(* Logix 5000 AddOnInstructionDefinition export YAI_Assy_166_115_EIP_Hz; software revision 21.03 *)

ADD_ON_INSTRUCTION YAI_Assy_166_115_EIP_Hz   (* revision 1.0, vendor Yaskawa America, Inc. *)
// YAI Assembly 166 and 115
// Help:
// This add-on instruction is for use with input assemblie 166 and output assemblies 115.
// Node_Input_Assy is defined as the node's input assembly integer array.
// Node_Output_Assy is defined as the node's output assembly integer array.
// Torque limit/reference, torque compensation and torque output variables are only available with A1000.
VAR_IN_OUT
   Node_Input_Assy : AB:ETHERNET_MODULE_INT_44Bytes:I:0; {required}   // Input assembly words
   Node_Output_Assy : AB:ETHERNET_MODULE_INT_40Bytes:O:0; {required}   // Output assembly words
END_VAR
VAR_INPUT
   RunFwd : BOOL; {visible}   // Forward run command
   RunRev : BOOL; {visible}   // Reverse run command
   MFI_3 : BOOL; {visible}   // Multi-function input 3
   MFI_4 : BOOL; {visible}   // Multi-function input 4
   MFI_5 : BOOL; {visible}   // Multi-function input 5
   MFI_6 : BOOL; {visible}   // Multi-function input 6
   MFI_7 : BOOL; {visible}   // Multi-function input 7
   MFI_8 : BOOL; {visible}   // Multi-function input 8
   External_Fault : BOOL;   // External fault command (EF0)
   FaultReset : BOOL; {visible}   // Fault reset command
   MFO_1 : BOOL; {visible}   // Multi-function output (M1-M2 for A/P1000, MA/MB/MC for V1000)
   MFO_2 : BOOL; {visible}   // Multi-function output (M3-M4 for A/P1000, P1 for V1000)
   MFO_3 : BOOL; {visible}   // Multi-function output (M5-M6 for A/P1000, P2 for V1000)
   Freq_Ref : REAL; {visible}   // Frequency reference command in Hz (xx.xx resolution)
   Torq_Ref_Limit : REAL; {visible}   // Torque reference/limit (A1000 only)
   Torq_Comp : REAL; {visible}   // Torque compensation command (A1000 only)
   Analog_Output_1 : REAL;   // Analog output 1 level command
   Analog_Output_2 : REAL;   // Analog output 2 level command
   Digital_Output_1 : BOOL;   // Digital output 1 activation - M1-M2
   Digital_Output_2 : BOOL;   // Digital output 2 activation - M3-M4
   Digital_Output_3 : BOOL;   // Digital output 3 activation - M5-M6
   Digital_Output_Fault_Enable : BOOL;   // Bit to enable control of fault output relay over the network
   Digital_Output_Fault : BOOL;   // Fault relay activation - MA-MB-MC
END_VAR
VAR_OUTPUT
   Alarm : BOOL; {access Read Only, visible}   // Drive alarm status bit
   Analog_Input_1_Level : REAL; {access Read Only}   // Analog input 1 level in % (xxx.x resolution)
   At_Speed : BOOL; {access Read Only, visible}   // Drive at commanded speed status bit
   Custom_In_1 : INT; {access Read Only, visible}   // Custom input 1 - F7-33
   Custom_In_1_Error : BOOL; {access Read Only}   // Custom input 1 error bit
   Custom_In_2 : INT; {access Read Only, visible}   // Custom input 2 - F7-34
   Custom_In_2_Error : BOOL; {access Read Only}   // Custom input 2 error bit
   Custom_In_3 : INT; {access Read Only, visible}   // Custom input 3 - F7-35
   Custom_In_3_Error : BOOL; {access Read Only}   // Custom input 3 error bit
   Custom_In_4 : INT; {access Read Only}   // Custom input 4 - F7-36
   Custom_In_4_Error : BOOL; {access Read Only}   // Custom input 4 error bit
   Custom_In_5 : INT; {access Read Only}   // Custom input 5 - F7-37
   Custom_In_5_Error : BOOL; {access Read Only}   // Custom input 5 error bit
   Custom_In_6 : INT; {access Read Only}   // Custom input 6 - F7-38
   Custom_In_6_Error : BOOL; {access Read Only}   // Custom input 6 error bit
   Custom_In_7 : INT; {access Read Only}   // Custom input 7 - F7-39
   Custom_In_7_Error : BOOL; {access Read Only}   // Custom input 7 error bit
   Custom_In_8 : INT; {access Read Only}   // Custom input 8 -F7-40
   Custom_In_8_Error : BOOL; {access Read Only}   // Custom input 8 error bit
   Custom_In_9 : INT; {access Read Only}   // Custom input 9 - F7-41
   Custom_In_9_Error : BOOL; {access Read Only}   // Custom input 9 error bit
   Custom_In_10 : INT; {access Read Only}   // Custom input 10 - F7-42
   Custom_In_10_Error : BOOL; {access Read Only}   // Custom input 10 error bit
   Custom_Out_1_Error : BOOL; {access Read Only}   // Custom output 1 error bit
   Custom_Out_2_Error : BOOL; {access Read Only}   // Custom output 2 error bit
   Custom_Out_3_Error : BOOL; {access Read Only}   // Custom output 3 error bit
   Custom_Out_4_Error : BOOL; {access Read Only}   // Custom output 4 error bit
   Custom_Out_5_Error : BOOL; {access Read Only}   // Custom output 5 error bit
   Custom_Out_6_Error : BOOL; {access Read Only}   // Custom output 6 error bit
   Custom_Out_7_Error : BOOL; {access Read Only}   // Custom output 7 error bit
   Custom_Out_8_Error : BOOL; {access Read Only}   // Custom output 8 error bit
   Custom_Out_9_Error : BOOL; {access Read Only}   // Custom output 9 error bit
   Custom_Out_10_Error : BOOL; {access Read Only}   // Custom output 10 error bit
   DC_Bus_Volt : INT; {access Read Only, visible}   // DC bus voltage in Vdc (xxx resolution)
   Error_Code : INT; {access Read Only}   // Custom input/output error code. Refer to custom error bit to determine which parameter error is pertaining to.
   Faulted : BOOL; {access Read Only, visible}   // Drive faulted status bit
   Freq_Cmd : REAL; {access Read Only, visible}   // Commanded frequency in Hz (xx.xx resolution)
   MFO_1_Status : BOOL; {access Read Only, visible}   // Drive multi-function output 1 (M1-M2 for A/P1000, MA/MB/MC for V1000) status
   MFO_2_Status : BOOL; {access Read Only, visible}   // Drive multi-function output 1 (M3-M4 for A/P1000, P1 for V1000) status
   MFO_3_Status : BOOL; {access Read Only, visible}   // Drive multi-function output 1 (M5-M6 for A/P1000, P2 for V1000) status
   Motor_Speed : REAL; {access Read Only, visible}   // Motor speed in Hz (xx.xx resolution)
   NetCtrlStatus : BOOL; {access Read Only, visible}   // Drive network run source status bit (1 = source coming from network)
   OPE : BOOL; {access Read Only}   // OPE alarm/fault present
   Output_Current : REAL; {access Read Only, visible}   // Drive output current in A (xxx.x resolution)
   Output_Freq : REAL; {access Read Only, visible}   // Drive output frequency in Hz (xx.xx resolution)
   PG_Count : INT; {access Read Only}   // Encoder feedback count
   Ready : BOOL; {access Read Only, visible}   // Drive ready status bit
   Reset : BOOL; {access Read Only, visible}   // Drive reset command status bit
   Running : BOOL; {access Read Only, visible}   // Drive running forward status bit
   RunningRev : BOOL; {access Read Only, visible}   // Drive running reverse status bit
   Torque_Actual : REAL; {access Read Only, visible}   // Drive torque output in % (xxx.x resolution)
   UV : BOOL; {access Read Only}   // Drive in UV (undervoltage) state status bit
   ZSP : BOOL; {access Read Only, visible}   // Drive zero speed status bit
   ZSV : BOOL; {access Read Only, visible}   // Drive zero servo completed status bit
END_VAR
VAR
   FRef_Convert : DINT;
   FOut_Convert : REAL;
   FOut_Temp : REAL;
   TRef_Convert : INT;
   TComp_Convert : INT;
   TOut_Convert : REAL;
   TOut_Temp : REAL;
   IOut_Temp : REAL;
   IOut_Convert : REAL;
   AO1_Convert : INT;
   AO2_Convert : INT;
   Motor_Speed_Temp : REAL;
   Motor_Speed_Convert : REAL;
   Freq_Cmd_Temp : REAL;
   Freq_Cmd_Convert : REAL;
   AI1_Temp : REAL;
   AI1_Convert : REAL;
   AI2_Temp : REAL; {access None}
   AI2_Convert : REAL; {access None}
   AI3_Temp : REAL; {access None}
   AI3_Convert : REAL; {access None}
END_VAR

ROUTINE Logic   (* ladder *)
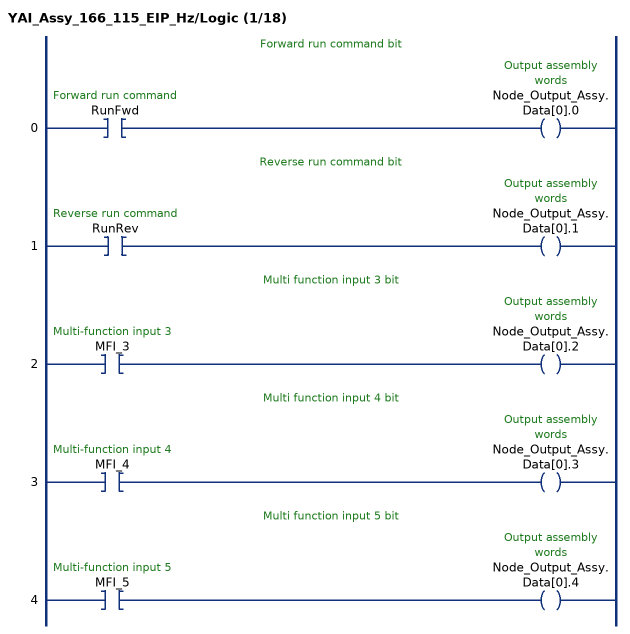
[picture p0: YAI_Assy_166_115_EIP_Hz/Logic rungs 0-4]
   // Forward run command bit
   0: XIC(RunFwd)OTE(Node_Output_Assy.Data[0].0);
   // Reverse run command bit
   1: XIC(RunRev)OTE(Node_Output_Assy.Data[0].1);
   // Multi function input 3 bit
   2: XIC(MFI_3)OTE(Node_Output_Assy.Data[0].2);
   // Multi function input 4 bit
   3: XIC(MFI_4)OTE(Node_Output_Assy.Data[0].3);
   // Multi function input 5 bit
   4: XIC(MFI_5)OTE(Node_Output_Assy.Data[0].4);
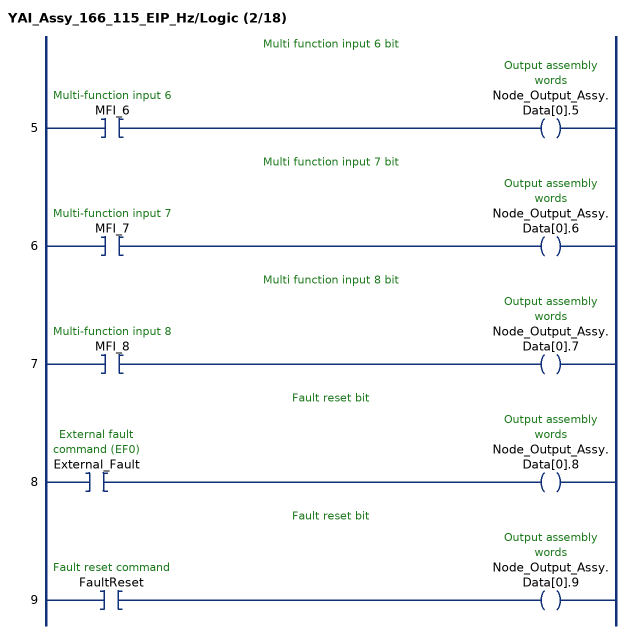
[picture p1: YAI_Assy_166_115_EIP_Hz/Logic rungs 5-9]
   // Multi function input 6 bit
   5: XIC(MFI_6)OTE(Node_Output_Assy.Data[0].5);
   // Multi function input 7 bit
   6: XIC(MFI_7)OTE(Node_Output_Assy.Data[0].6);
   // Multi function input 8 bit
   7: XIC(MFI_8)OTE(Node_Output_Assy.Data[0].7);
   // Fault reset bit
   8: XIC(External_Fault)OTE(Node_Output_Assy.Data[0].8);
   // Fault reset bit
   9: XIC(FaultReset)OTE(Node_Output_Assy.Data[0].9);
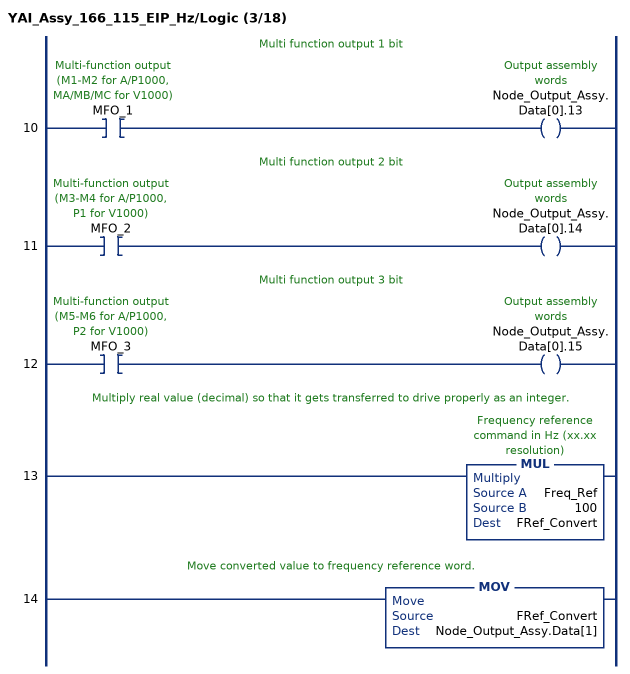
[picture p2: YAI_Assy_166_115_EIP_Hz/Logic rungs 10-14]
   // Multi function output 1 bit
   10: XIC(MFO_1)OTE(Node_Output_Assy.Data[0].13);
   // Multi function output 2 bit
   11: XIC(MFO_2)OTE(Node_Output_Assy.Data[0].14);
   // Multi function output 3 bit
   12: XIC(MFO_3)OTE(Node_Output_Assy.Data[0].15);
   // Multiply real value (decimal) so that it gets transferred to drive properly as an integer.
   13: MUL(Freq_Ref,100,FRef_Convert);
   // Move converted value to frequency reference word.
   14: MOV(FRef_Convert,Node_Output_Assy.Data[1]);
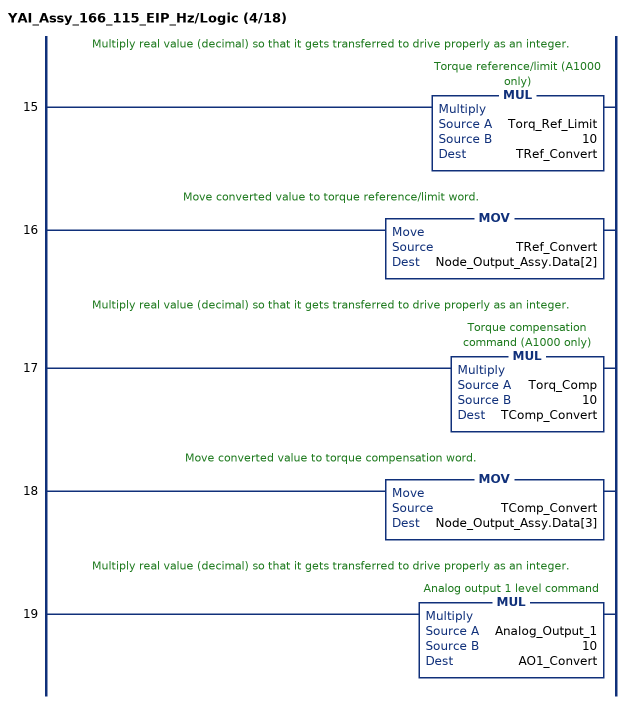
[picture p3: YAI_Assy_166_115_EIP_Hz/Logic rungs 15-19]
   // Multiply real value (decimal) so that it gets transferred to drive properly as an integer.
   15: MUL(Torq_Ref_Limit,10,TRef_Convert);
   // Move converted value to torque reference/limit word.
   16: MOV(TRef_Convert,Node_Output_Assy.Data[2]);
   // Multiply real value (decimal) so that it gets transferred to drive properly as an integer.
   17: MUL(Torq_Comp,10,TComp_Convert);
   // Move converted value to torque compensation word.
   18: MOV(TComp_Convert,Node_Output_Assy.Data[3]);
   // Multiply real value (decimal) so that it gets transferred to drive properly as an integer.
   19: MUL(Analog_Output_1,10,AO1_Convert);
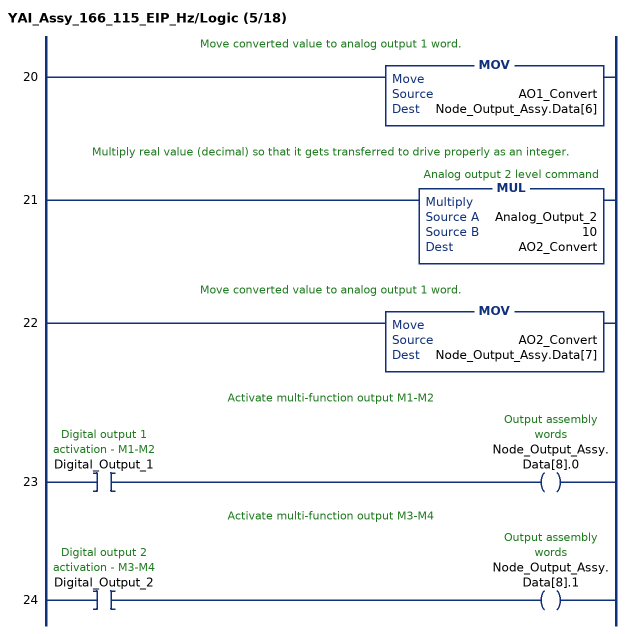
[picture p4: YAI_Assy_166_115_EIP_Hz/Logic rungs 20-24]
   // Move converted value to analog output 1 word.
   20: MOV(AO1_Convert,Node_Output_Assy.Data[6]);
   // Multiply real value (decimal) so that it gets transferred to drive properly as an integer.
   21: MUL(Analog_Output_2,10,AO2_Convert);
   // Move converted value to analog output 1 word.
   22: MOV(AO2_Convert,Node_Output_Assy.Data[7]);
   // Activate multi-function output M1-M2
   23: XIC(Digital_Output_1)OTE(Node_Output_Assy.Data[8].0);
   // Activate multi-function output M3-M4
   24: XIC(Digital_Output_2)OTE(Node_Output_Assy.Data[8].1);
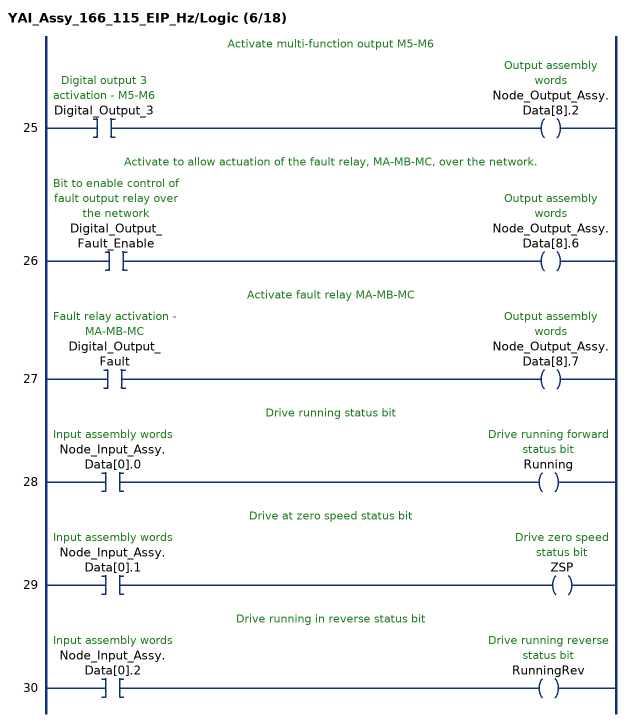
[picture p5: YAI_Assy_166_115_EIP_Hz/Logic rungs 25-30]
   // Activate multi-function output M5-M6
   25: XIC(Digital_Output_3)OTE(Node_Output_Assy.Data[8].2);
   // Activate to allow actuation of the fault relay, MA-MB-MC, over the network.
   26: XIC(Digital_Output_Fault_Enable)OTE(Node_Output_Assy.Data[8].6);
   // Activate fault relay MA-MB-MC
   27: XIC(Digital_Output_Fault)OTE(Node_Output_Assy.Data[8].7);
   // Drive running status bit
   28: XIC(Node_Input_Assy.Data[0].0)OTE(Running);
   // Drive at zero speed status bit
   29: XIC(Node_Input_Assy.Data[0].1)OTE(ZSP);
   // Drive running in reverse status bit
   30: XIC(Node_Input_Assy.Data[0].2)OTE(RunningRev);
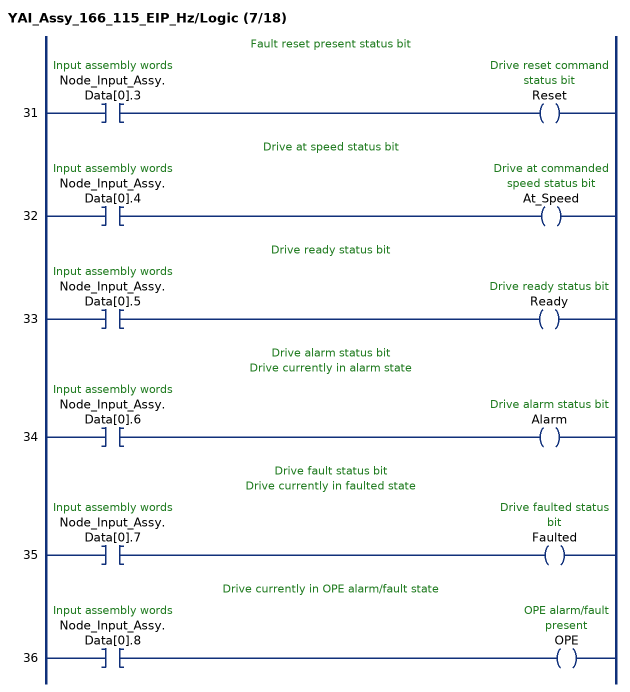
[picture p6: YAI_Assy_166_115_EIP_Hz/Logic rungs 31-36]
   // Fault reset present status bit
   31: XIC(Node_Input_Assy.Data[0].3)OTE(Reset);
   // Drive at speed status bit
   32: XIC(Node_Input_Assy.Data[0].4)OTE(At_Speed);
   // Drive ready status bit
   33: XIC(Node_Input_Assy.Data[0].5)OTE(Ready);
   // Drive alarm status bit
   // Drive currently in alarm state
   34: XIC(Node_Input_Assy.Data[0].6)OTE(Alarm);
   // Drive fault status bit
   // Drive currently in faulted state
   35: XIC(Node_Input_Assy.Data[0].7)OTE(Faulted);
   // Drive currently in OPE alarm/fault state
   36: XIC(Node_Input_Assy.Data[0].8)OTE(OPE);
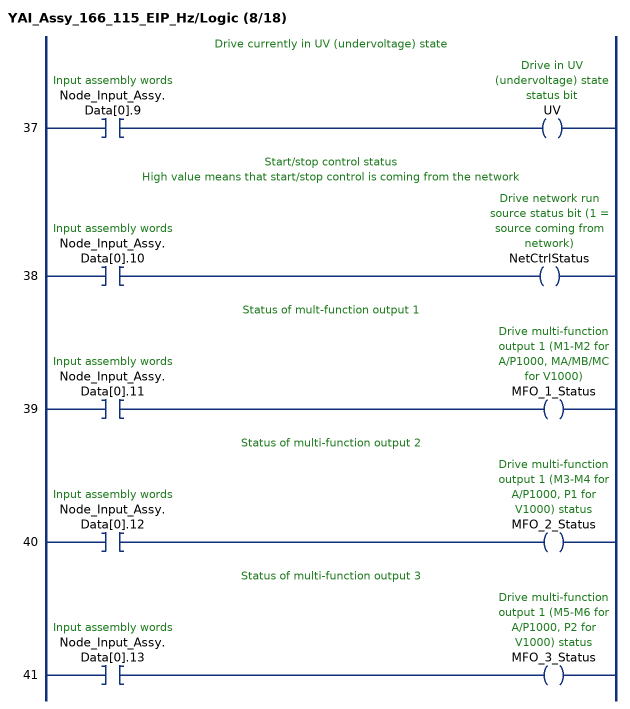
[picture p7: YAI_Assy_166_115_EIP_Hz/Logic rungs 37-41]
   // Drive currently in UV (undervoltage) state
   37: XIC(Node_Input_Assy.Data[0].9)OTE(UV);
   // Start/stop control status
   // High value means that start/stop control is coming from the network
   38: XIC(Node_Input_Assy.Data[0].10)OTE(NetCtrlStatus);
   // Status of mult-function output 1
   39: XIC(Node_Input_Assy.Data[0].11)OTE(MFO_1_Status);
   // Status of multi-function output 2
   40: XIC(Node_Input_Assy.Data[0].12)OTE(MFO_2_Status);
   // Status of multi-function output 3
   41: XIC(Node_Input_Assy.Data[0].13)OTE(MFO_3_Status);
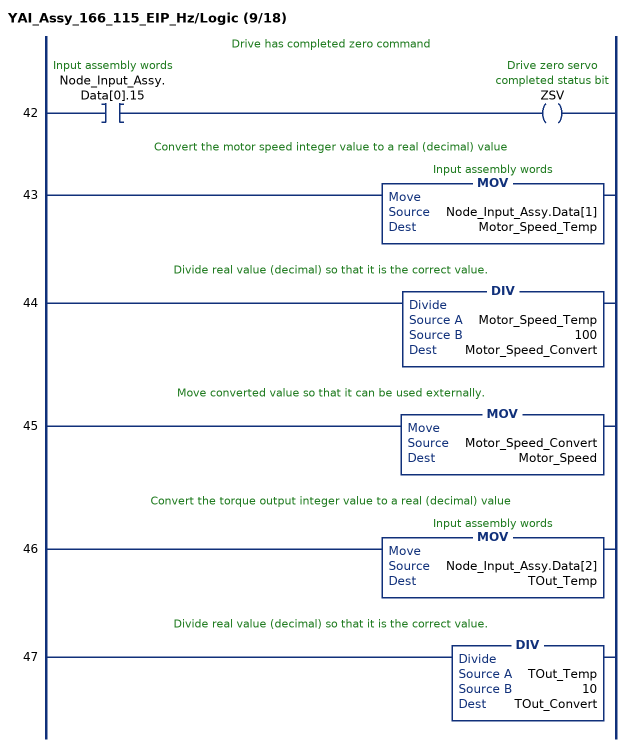
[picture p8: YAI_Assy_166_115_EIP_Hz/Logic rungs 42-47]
   // Drive has completed zero command
   42: XIC(Node_Input_Assy.Data[0].15)OTE(ZSV);
   // Convert the motor speed integer value to a real (decimal) value
   43: MOV(Node_Input_Assy.Data[1],Motor_Speed_Temp);
   // Divide real value (decimal) so that it is the correct value.
   44: DIV(Motor_Speed_Temp,100,Motor_Speed_Convert);
   // Move converted value so that it can be used externally.
   45: MOV(Motor_Speed_Convert,Motor_Speed);
   // Convert the torque output integer value to a real (decimal) value
   46: MOV(Node_Input_Assy.Data[2],TOut_Temp);
   // Divide real value (decimal) so that it is the correct value.
   47: DIV(TOut_Temp,10,TOut_Convert);
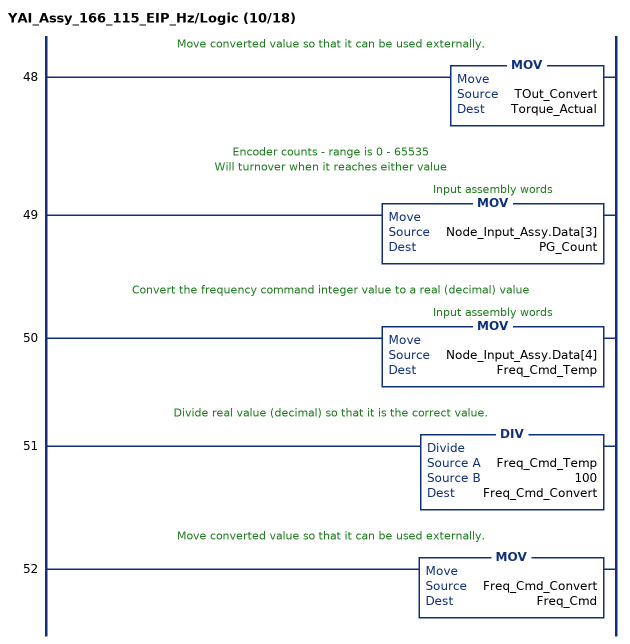
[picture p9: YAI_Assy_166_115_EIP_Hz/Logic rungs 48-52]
   // Move converted value so that it can be used externally.
   48: MOV(TOut_Convert,Torque_Actual);
   // Encoder counts - range is 0 - 65535
   // Will turnover when it reaches either value
   49: MOV(Node_Input_Assy.Data[3],PG_Count);
   // Convert the frequency command integer value to a real (decimal) value
   50: MOV(Node_Input_Assy.Data[4],Freq_Cmd_Temp);
   // Divide real value (decimal) so that it is the correct value.
   51: DIV(Freq_Cmd_Temp,100,Freq_Cmd_Convert);
   // Move converted value so that it can be used externally.
   52: MOV(Freq_Cmd_Convert,Freq_Cmd);
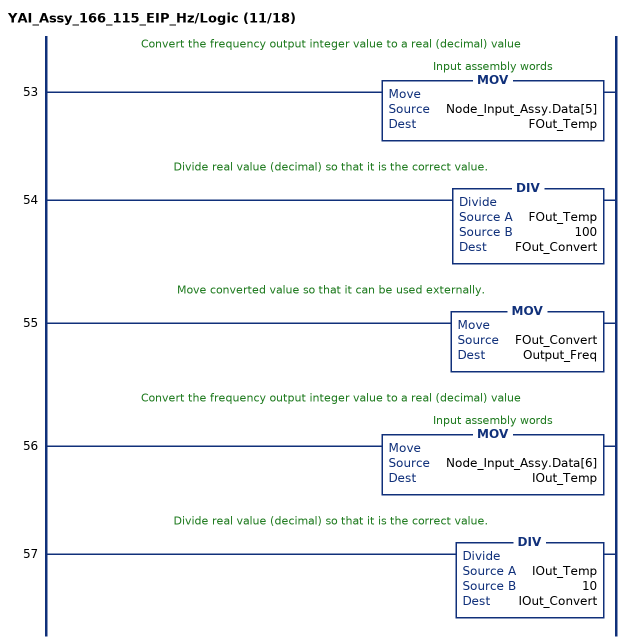
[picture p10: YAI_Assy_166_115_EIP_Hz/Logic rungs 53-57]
   // Convert the frequency output integer value to a real (decimal) value
   53: MOV(Node_Input_Assy.Data[5],FOut_Temp);
   // Divide real value (decimal) so that it is the correct value.
   54: DIV(FOut_Temp,100,FOut_Convert);
   // Move converted value so that it can be used externally.
   55: MOV(FOut_Convert,Output_Freq);
   // Convert the frequency output integer value to a real (decimal) value
   56: MOV(Node_Input_Assy.Data[6],IOut_Temp);
   // Divide real value (decimal) so that it is the correct value.
   57: DIV(IOut_Temp,10,IOut_Convert);
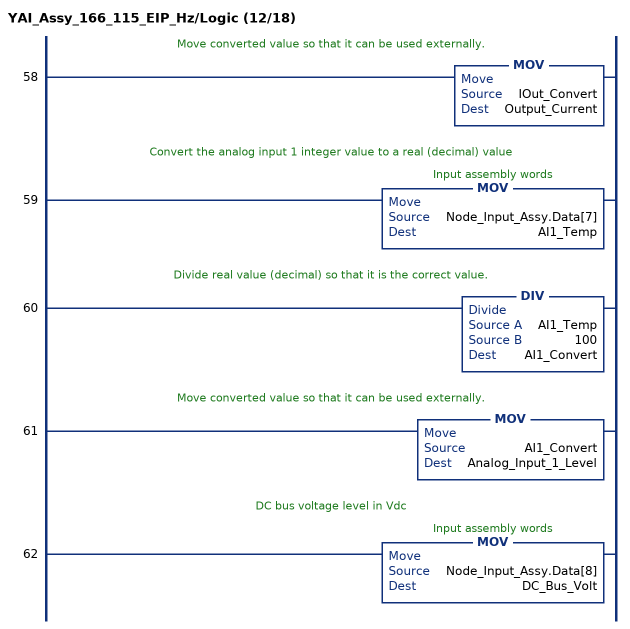
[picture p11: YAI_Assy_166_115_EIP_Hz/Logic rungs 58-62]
   // Move converted value so that it can be used externally.
   58: MOV(IOut_Convert,Output_Current);
   // Convert the analog input 1 integer value to a real (decimal) value
   59: MOV(Node_Input_Assy.Data[7],AI1_Temp);
   // Divide real value (decimal) so that it is the correct value.
   60: DIV(AI1_Temp,100,AI1_Convert);
   // Move converted value so that it can be used externally.
   61: MOV(AI1_Convert,Analog_Input_1_Level);
   // DC bus voltage level in Vdc
   62: MOV(Node_Input_Assy.Data[8],DC_Bus_Volt);
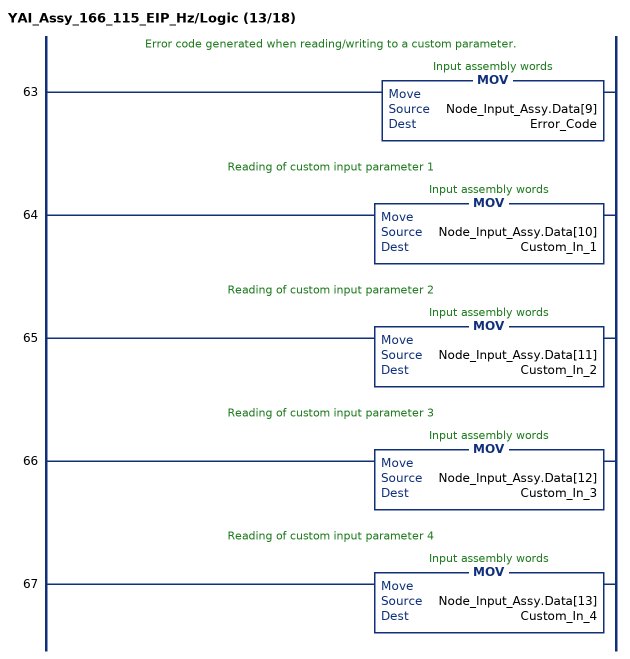
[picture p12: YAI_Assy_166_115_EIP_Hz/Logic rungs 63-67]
   // Error code generated when reading/writing to a custom parameter.
   63: MOV(Node_Input_Assy.Data[9],Error_Code);
   // Reading of custom input parameter 1
   64: MOV(Node_Input_Assy.Data[10],Custom_In_1);
   // Reading of custom input parameter 2
   65: MOV(Node_Input_Assy.Data[11],Custom_In_2);
   // Reading of custom input parameter 3
   66: MOV(Node_Input_Assy.Data[12],Custom_In_3);
   // Reading of custom input parameter 4
   67: MOV(Node_Input_Assy.Data[13],Custom_In_4);
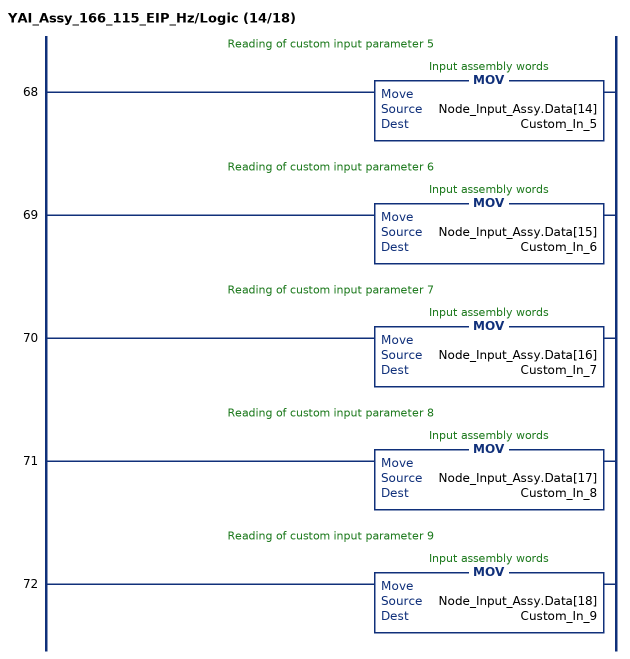
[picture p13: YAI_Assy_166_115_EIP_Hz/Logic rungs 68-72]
   // Reading of custom input parameter 5
   68: MOV(Node_Input_Assy.Data[14],Custom_In_5);
   // Reading of custom input parameter 6
   69: MOV(Node_Input_Assy.Data[15],Custom_In_6);
   // Reading of custom input parameter 7
   70: MOV(Node_Input_Assy.Data[16],Custom_In_7);
   // Reading of custom input parameter 8
   71: MOV(Node_Input_Assy.Data[17],Custom_In_8);
   // Reading of custom input parameter 9
   72: MOV(Node_Input_Assy.Data[18],Custom_In_9);
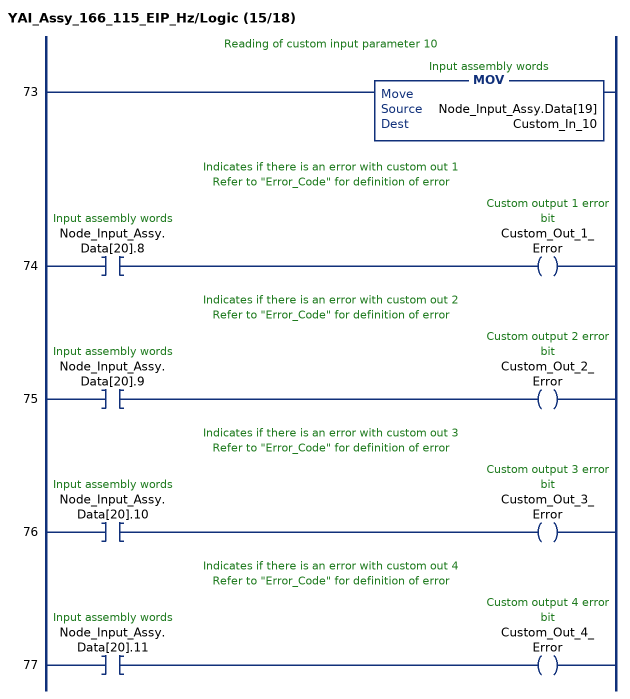
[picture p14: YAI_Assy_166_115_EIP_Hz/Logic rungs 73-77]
   // Reading of custom input parameter 10
   73: MOV(Node_Input_Assy.Data[19],Custom_In_10);
   // Indicates if there is an error with custom out 1
   // Refer to "Error_Code" for definition of error
   74: XIC(Node_Input_Assy.Data[20].8)OTE(Custom_Out_1_Error);
   // Indicates if there is an error with custom out 2
   // Refer to "Error_Code" for definition of error
   75: XIC(Node_Input_Assy.Data[20].9)OTE(Custom_Out_2_Error);
   // Indicates if there is an error with custom out 3
   // Refer to "Error_Code" for definition of error
   76: XIC(Node_Input_Assy.Data[20].10)OTE(Custom_Out_3_Error);
   // Indicates if there is an error with custom out 4
   // Refer to "Error_Code" for definition of error
   77: XIC(Node_Input_Assy.Data[20].11)OTE(Custom_Out_4_Error);
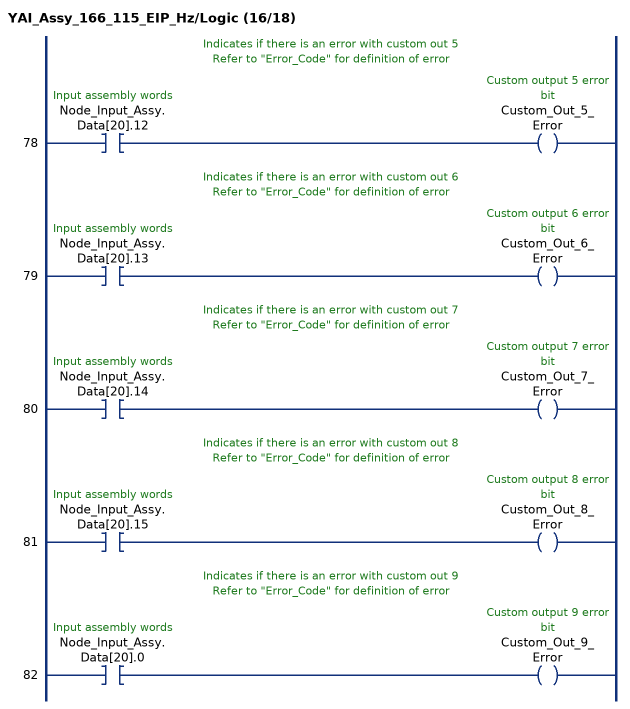
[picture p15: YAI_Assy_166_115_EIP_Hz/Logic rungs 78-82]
   // Indicates if there is an error with custom out 5
   // Refer to "Error_Code" for definition of error
   78: XIC(Node_Input_Assy.Data[20].12)OTE(Custom_Out_5_Error);
   // Indicates if there is an error with custom out 6
   // Refer to "Error_Code" for definition of error
   79: XIC(Node_Input_Assy.Data[20].13)OTE(Custom_Out_6_Error);
   // Indicates if there is an error with custom out 7
   // Refer to "Error_Code" for definition of error
   80: XIC(Node_Input_Assy.Data[20].14)OTE(Custom_Out_7_Error);
   // Indicates if there is an error with custom out 8
   // Refer to "Error_Code" for definition of error
   81: XIC(Node_Input_Assy.Data[20].15)OTE(Custom_Out_8_Error);
   // Indicates if there is an error with custom out 9
   // Refer to "Error_Code" for definition of error
   82: XIC(Node_Input_Assy.Data[20].0)OTE(Custom_Out_9_Error);
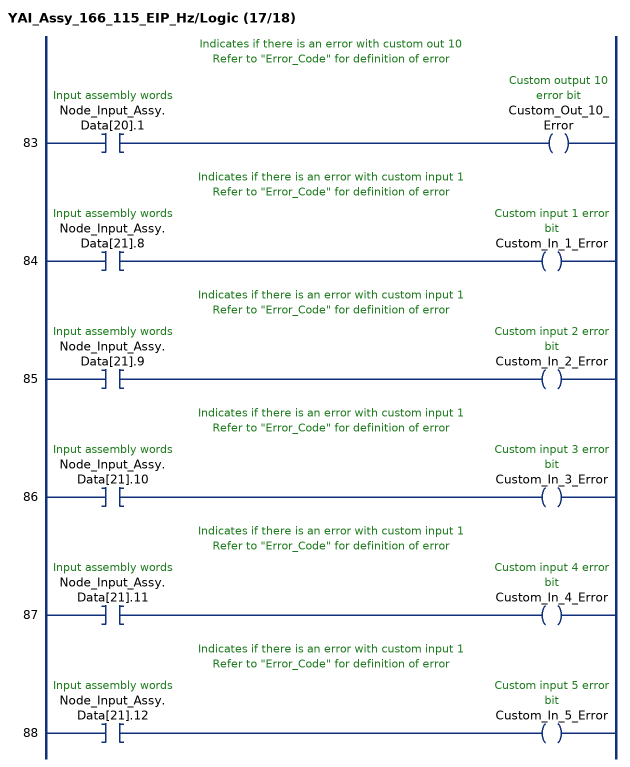
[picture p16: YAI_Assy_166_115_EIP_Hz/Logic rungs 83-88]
   // Indicates if there is an error with custom out 10
   // Refer to "Error_Code" for definition of error
   83: XIC(Node_Input_Assy.Data[20].1)OTE(Custom_Out_10_Error);
   // Indicates if there is an error with custom input 1
   // Refer to "Error_Code" for definition of error
   84: XIC(Node_Input_Assy.Data[21].8)OTE(Custom_In_1_Error);
   // Indicates if there is an error with custom input 1
   // Refer to "Error_Code" for definition of error
   85: XIC(Node_Input_Assy.Data[21].9)OTE(Custom_In_2_Error);
   // Indicates if there is an error with custom input 1
   // Refer to "Error_Code" for definition of error
   86: XIC(Node_Input_Assy.Data[21].10)OTE(Custom_In_3_Error);
   // Indicates if there is an error with custom input 1
   // Refer to "Error_Code" for definition of error
   87: XIC(Node_Input_Assy.Data[21].11)OTE(Custom_In_4_Error);
   // Indicates if there is an error with custom input 1
   // Refer to "Error_Code" for definition of error
   88: XIC(Node_Input_Assy.Data[21].12)OTE(Custom_In_5_Error);
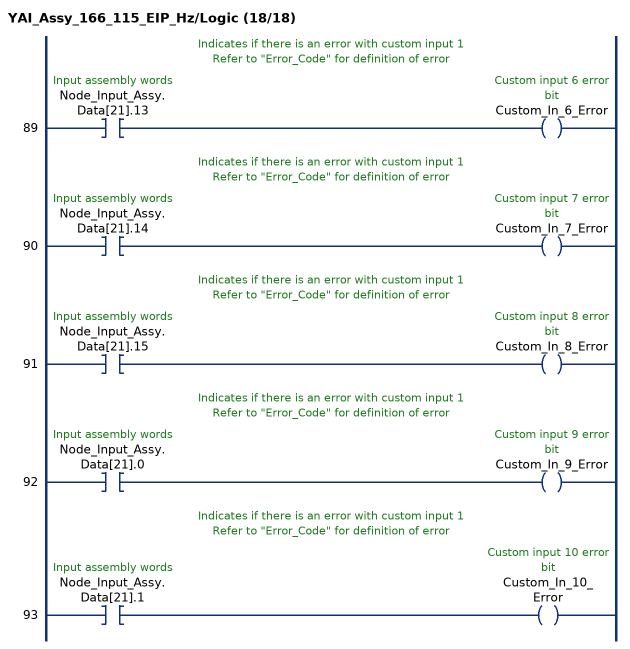
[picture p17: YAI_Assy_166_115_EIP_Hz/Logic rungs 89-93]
   // Indicates if there is an error with custom input 1
   // Refer to "Error_Code" for definition of error
   89: XIC(Node_Input_Assy.Data[21].13)OTE(Custom_In_6_Error);
   // Indicates if there is an error with custom input 1
   // Refer to "Error_Code" for definition of error
   90: XIC(Node_Input_Assy.Data[21].14)OTE(Custom_In_7_Error);
   // Indicates if there is an error with custom input 1
   // Refer to "Error_Code" for definition of error
   91: XIC(Node_Input_Assy.Data[21].15)OTE(Custom_In_8_Error);
   // Indicates if there is an error with custom input 1
   // Refer to "Error_Code" for definition of error
   92: XIC(Node_Input_Assy.Data[21].0)OTE(Custom_In_9_Error);
   // Indicates if there is an error with custom input 1
   // Refer to "Error_Code" for definition of error
   93: XIC(Node_Input_Assy.Data[21].1)OTE(Custom_In_10_Error);
END_ROUTINE
END_ADD_ON_INSTRUCTION
